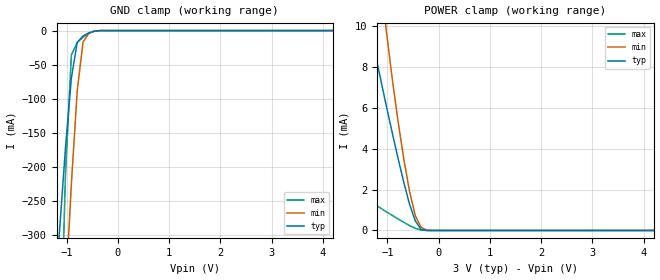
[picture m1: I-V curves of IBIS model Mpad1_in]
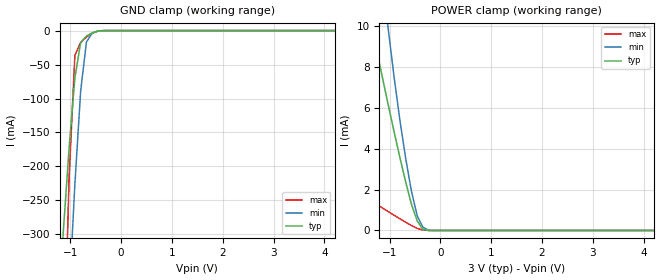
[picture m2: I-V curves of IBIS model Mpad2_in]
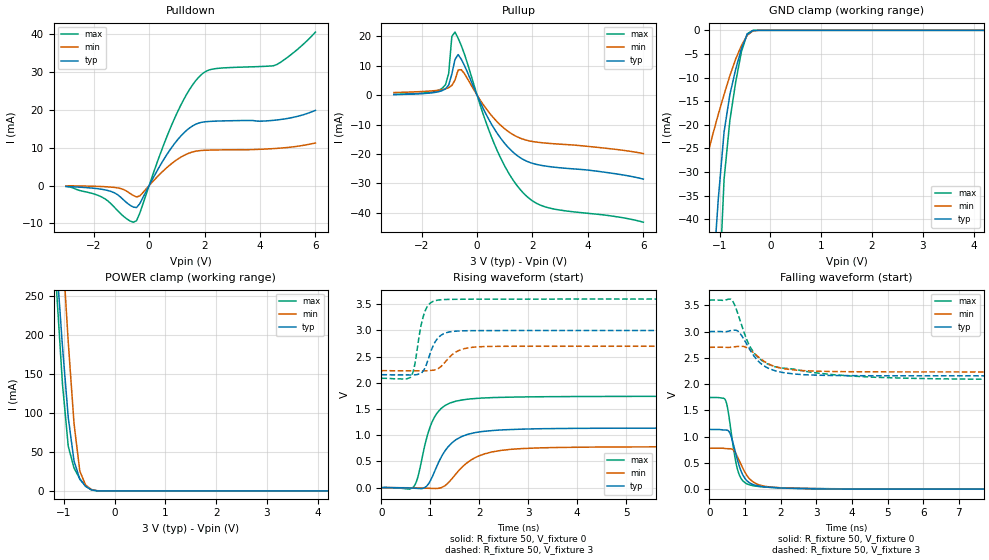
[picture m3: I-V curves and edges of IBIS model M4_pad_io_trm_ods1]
| Created by SiliconSmart  O-2018.09-SP2-3
[IBIS Ver]   4.0
[File Name]   as3316tb_rev1p3.ibs
[File Rev]   1.3
[Date]   Thursday Mar 21 2024
|[Source]   Avalanche Team
|[Notes]   Generated IBIS models from Silicon Smart
|[Rev 1.0]  Initial Release based on extracted netlist
|   Characterization
|[Rev 1.1]  Recharacterization with Hspice, run in high accuracy mode
|[Rev 1.2]  Recharacterization with Hspice, align with parameters
|   in datasheet rev T
|[Rev 1.3]  Update the pin to the package pinout assignment
|[Disclaimer]   THE MODEL LIBRARIES ARE PROVIDED AS IS.
|[Copyright]   Copyright 2019, Avalanche Technology., All Rights Reserved
[Component]   as30xx316_TSOP54
[Manufacturer] Avalanche Technology
| CONTENT :
| This file contains IBIS MODEL for PSRAM device
| AS3032316
| USAGE :
| The models are derived for the 2.7V to 3.6V I/O Operation.
| Temperatures for model generation: typ: 25, max: -40, min: 105
| Voltages : typ: 3.0V, min: 2.7V, max: 3.6V
| PACKAGES SUPPORTED :
| 54-pin TSOP (10mm x 22mm)
| VERIFICATION
| Errors  : 0
| Warnings: 11
| All warnings due to non-monotonic data:
[Package]
R_pkg   0   0 0
L_pkg   0   0 0
C_pkg   0   0 0
[Pin]   signal_name   model_name R_pin   L_pin   C_pin
1   ADDR_20   Mpad1_in   0.242	9.288E-9	1.318E-12
2   ADDR_19   Mpad1_in   0.230	8.645E-9	1.393E-12
3   ADDR_0   Mpad1_in   0.220	8.000E-9	1.249E-12
4   ADDR_1   Mpad1_in   0.202	7.235E-9	1.120E-12
5   ADDR_2   Mpad1_in   0.190	6.504E-9	9.932E-13
6   ADDR_3   Mpad1_in   0.183	5.790E-9	7.992E-13
7   ADDR_4   Mpad1_in   0.153	4.971E-9	7.183E-13
8   E#   Mpad2_in   0.144	4.305E-9	7.146E-13
9   DQ_0   Mpad_io   0.133	3.895E-9	6.207E-13
10   DQ_1   Mpad_io   0.123	3.499E-9	5.802E-13
11   DQ_2   Mpad_io   0.118	3.169E-9	5.261E-13
12   DQ_3   Mpad_io   0.114	2.900E-9	4.467E-13
15   DQ_4   Mpad_io   0.109	2.671E-9	4.016E-13
16   DQ_5   Mpad_io   0.111	2.843E-9	4.439E-13
17   DQ_6   Mpad_io   0.114	3.087E-9	5.185E-13
18   DQ_7   Mpad_io   0.118	3.390E-9	5.728E-13
19   W#   Mpad2_in   0.125	3.746E-9	6.059E-13
20   ADDR_5   Mpad1_in   0.134	4.125E-9	6.880E-13
21   ADDR_6   Mpad1_in   0.156	5.043E-9	7.141E-13
22   ADDR_7   Mpad1_in   0.191	5.914E-9	8.117E-13
23   ADDR_8   Mpad1_in   0.203	6.653E-9	1.003E-12
24   ADDR_9   Mpad1_in   0.215	7.410E-9	1.094E-12
31   ADDR_10   Mpad1_in   0.215	7.409E-9	1.099E-12
32   ADDR_11   Mpad1_in   0.202	6.635E-9	1.007E-12
33   ADDR_12   Mpad1_in   0.190	5.904E-9	8.154E-13
34   ADDR_13   Mpad1_in   0.155	5.033E-9	7.165E-13
35   ADDR_14   Mpad1_in   0.134	4.125E-9	6.860E-13
37   DQ_8   Mpad_io   0.118	3.397E-9	5.722E-13
38   DQ_9   Mpad_io   0.114	3.090E-9	5.214E-13
39   DQ_10   Mpad_io   0.111	2.837E-9	4.444E-13
40   DQ_11   Mpad_io   0.109	2.663E-9	4.035E-13
43   DQ_12   Mpad_io   0.114	2.913E-9	4.507E-13
44   DQ_13   Mpad_io   0.118	3.178E-9	5.252E-13
45   DQ_14   Mpad_io   0.123	3.501E-9	5.817E-13
46   DQ_15   Mpad_io   0.133	3.900E-9	6.217E-13
47   LB#   Mpad2_in   0.143	4.301E-9	7.117E-13
48   UB#   Mpad2_in   0.153	4.972E-9	7.207E-13
49   G#   Mpad2_in   0.179	5.774E-9	7.991E-13
50   ADDR_15   Mpad1_in   0.191	6.496E-9	9.963E-13
51   ADDR_16   Mpad1_in   0.204	7.263E-9	1.127E-12
52   ADDR_17   Mpad1_in   0.221	8.012E-9	1.250E-12
53   ADDR_18   Mpad1_in   0.232	8.680E-9	1.364E-12
13   VCC   POWER   NA   NA   NA
14   VSS   GND   NA   NA   NA
41   VCC   POWER   NA   NA   NA
42   VSS   GND   NA   NA   NA
| pad_io
[Model Selector] Mpad_io
| Model Description
M4_pad_io_trm_ods1   60 Ohms drv strength
| Models and submodels in the file (3): Mpad1_in (Input), Mpad2_in (Input), M4_pad_io_trm_ods1 (I/O)
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| pad1_in
[Model] Mpad1_in
Model_type Input
Enable   Active-High
Vinl  =  0.6
Vinh  =  2.4
| Capacitance  typ   min   max
C_comp   2.857182e-12   2.353202e-12   3.152994e-12
| Variables   typ   min   max
[GND Clamp Reference]   0   0   0
[POWER Clamp Reference]   3   2.7   3.6
[Pulldown Reference]   0   0   0
[Pullup Reference]   3   2.7   3.6
[Temperature Range]   25   105   -40
[Voltage Range]   3   2.7   3.6
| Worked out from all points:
|   GND clamp passes 1 mA (typ) near -0.47 V on its own axis
|   POWER clamp passes 1 mA (typ) near -0.53 V on its own axis
[GND Clamp]
| Voltage   I(typ)   I(min)   I(max)
-3V       -2.489A    -3.622A    -6.286A
-1.252V   -415.1mA   -737.7mA   -841.9mA
-1.138V   -289.6mA   -559.5mA   -509.9mA
-1.024V   -170.9mA   -387mA     -208.5mA
-910.3mV  -69.58mA   -225.3mA   -35.91mA
-796.6mV  -17.5mA    -88.85mA   -17.44mA
-682.8mV  -8.077mA   -16.84mA   -9.651mA
-569mV    -3.425mA   -3.886mA   -3.679mA
-455.2mV  -663.4uA   -928.9uA   -526.9uA
-227.6mV  -421.5nA   -3.52uA    -35.99nA
6V        0A         0A         0A
[POWER Clamp]
| Voltage   I(typ)   I(min)   I(max)
-3V       32.41mA    56.72mA    4.109mA
-1.366V   10.2mA     17.4mA     1.461mA
-1.252V   8.822mA    14.8mA     1.281mA
-1.024V   6.137mA    9.837mA    922.9uA
-910.3mV  4.838mA    7.526mA    746.6uA
-796.6mV  3.581mA    5.417mA    573.1uA
-682.8mV  2.387mA    3.545mA    403.9uA
-569mV    1.291mA    1.93mA     242.9uA
-455.2mV  467.9uA    721.2uA    103.5uA
-341.4mV  48.97uA    156.2uA    20.84uA
-113.8mV  7.993nA    354.4nA    880.4pA
6V        0A         0A         0A
| pad2_in
[Model] Mpad2_in
Model_type Input
Enable   Active-High
Vinl  =  0.6
Vinh  =  2.4
| Capacitance  typ   min   max
C_comp   2.865723e-12   2.362138e-12   3.161751e-12
| Variables   typ   min   max
[GND Clamp Reference]   0   0   0
[POWER Clamp Reference]   3   2.7   3.6
[Pulldown Reference]   0   0   0
[Pullup Reference]   3   2.7   3.6
[Temperature Range]   25   105   -40
[Voltage Range]   3   2.7   3.6
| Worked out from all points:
|   GND clamp passes 1 mA (typ) near -0.47 V on its own axis
|   POWER clamp passes 1 mA (typ) near -0.53 V on its own axis
[GND Clamp]
| Voltage   I(typ)   I(min)   I(max)
-3V       -2.583A    -3.873A    -6.564A
-1.138V   -296.1mA   -573.1mA   -531mA
-1.024V   -173.3mA   -391.8mA   -216.6mA
-910.3mV  -69.77mA   -226.3mA   -36.44mA
-796.6mV  -17.49mA   -89.03mA   -17.43mA
-682.8mV  -8.073mA   -16.84mA   -9.646mA
-569mV    -3.423mA   -3.884mA   -3.677mA
-455.2mV  -662.9uA   -928.4uA   -526.4uA
-227.6mV  -421nA     -3.517uA   -35.92nA
6V        0A         0A         0A
[POWER Clamp]
| Voltage   I(typ)   I(min)   I(max)
-3V       32.41mA    56.72mA    4.109mA
-1.366V   10.2mA     17.4mA     1.461mA
-1.252V   8.822mA    14.8mA     1.281mA
-1.024V   6.137mA    9.837mA    922.9uA
-910.3mV  4.838mA    7.526mA    746.6uA
-796.6mV  3.581mA    5.417mA    573.1uA
-682.8mV  2.387mA    3.545mA    403.9uA
-569mV    1.291mA    1.93mA     242.9uA
-455.2mV  467.9uA    721.2uA    103.5uA
-341.4mV  48.97uA    156.2uA    20.84uA
-113.8mV  7.993nA    354.4nA    880.4pA
6V        0A         0A         0A
[Model] M4_pad_io_trm_ods1
Model_type I/O
Enable   Active-High
Vinl  =  0.6
Vinh  =  2.4
Vmeas =  1.5
Cref  =  30e-12
| Capacitance  typ   min   max
C_comp   4.118801e-12   3.947848e-12   4.414159e-12
| Variables   typ   min   max
[GND Clamp Reference]   0   0   0
[POWER Clamp Reference]   3   2.7   3.6
[Pulldown Reference]   0   0   0
[Pullup Reference]   3   2.7   3.6
[Temperature Range]   25   105   -40
[Voltage Range]   3   2.7   3.6
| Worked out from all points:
|   slope of the pulldown table from 0 to 0.45 V, typ, clamps not added: 75.6 ohm
|   slope of the pullup table from 0 to 0.45 V, typ, clamps not added: 51.8 ohm
|   GND clamp passes 1 mA (typ) near -0.46 V on its own axis
|   POWER clamp passes 1 mA (typ) near -0.42 V on its own axis
|   falling waveform, R_fixture 50, V_fixture 0: 20-80 % time 325ps typ, 411ps min, 252ps max; typ from 1.14 V to 0 V
|   falling waveform, R_fixture 50, V_fixture 3: 20-80 % time 602ps typ, 661ps min, 794ps max; typ from 3 V to 2.15 V
|   rising waveform, R_fixture 50, V_fixture 0: 20-80 % time 466ps typ, 621ps min, 335ps max; typ from 0 V to 1.14 V
|   rising waveform, R_fixture 50, V_fixture 3: 20-80 % time 225ps typ, 326ps min, 176ps max; typ from 2.15 V to 3 V
[GND Clamp]
| Voltage   I(typ)   I(min)   I(max)
-3V       -379.8mA   -106mA     -725.8mA
-1.593V   -131.7mA   -42.01mA   -247mA
-1.479V   -111.8mA   -36.94mA   -208.5mA
-1.138V   -53.52mA   -22.25mA   -94.22mA
-1.024V   -35.67mA   -17.76mA   -59.08mA
-910.3mV  -21.49mA   -13.58mA   -31.51mA
-796.6mV  -13.6mA    -9.604mA   -19.09mA
-682.8mV  -8.279mA   -6.099mA   -11mA
-569mV    -3.88mA    -3.236mA   -4.53mA
-455.2mV  -866.7uA   -1.043mA   -727.1uA
-341.4mV  -35.72uA   -109.2uA   -11.2uA
6V        0A         0A         0A
[POWER Clamp]
| Voltage   I(typ)   I(min)   I(max)
-3V       2.191A     2.679A     2.475A
-1.138V   291mA      439mA      255.8mA
-1.024V   186.1mA    312.2mA    137.6mA
-910.3mV  94.47mA    191.5mA    57.5mA
-796.6mV  38.47mA    86.67mA    29.42mA
-682.8mV  15.04mA    25.47mA    15.61mA
-569mV    5.939mA    7.524mA    6.125mA
-455.2mV  1.483mA    1.86mA     1.35mA
-227.6mV  1.148uA    12.93uA    332nA
6V        0A         0A         0A
[Pulldown]
| Voltage   I(typ)   I(min)   I(max)
-3V       -248.9uA   -57.27uA   -211.8uA
-1.934V   -763.9uA   -203.6uA   -2.351mA
-1.479V   -1.326mA   -352.6uA   -4.122mA
-796.6mV  -4.614mA   -1.551mA   -8.859mA
-455.2mV  -5.81mA    -3.008mA   -9.281mA
413.8mV   5.511mA    3.198mA    8.617mA
827.6mV   10.2mA     5.892mA    16.24mA
1.345V    14.53mA    8.266mA    23.98mA
1.759V    16.42mA    9.161mA    28.37mA
2.276V    16.97mA    9.375mA    30.72mA
4.614V    17.32mA    9.818mA    31.97mA
6V        19.86mA    11.25mA    40.51mA
[Pullup]
| Voltage   I(typ)   I(min)   I(max)
-3V       187.4uA    871.4uA    220.3uA
-1.252V   1.555mA    1.876mA    2.377mA
-1.024V   3.43mA     2.541mA    7.364mA
-910.3mV  7.139mA    3.267mA    19.92mA
-796.6mV  12.13mA    5.096mA    21.41mA
-682.8mV  13.76mA    8.544mA    19.32mA
-569mV    12.16mA    8.636mA    16.81mA
620.7mV   -11.43mA   -8.01mA    -16.55mA
1.138V    -17.91mA   -12.44mA   -26.44mA
1.655V    -21.81mA   -14.96mA   -33.11mA
2.586V    -24.25mA   -16.39mA   -38.3mA
6V        -28.52mA   -19.85mA   -43.17mA
[Ramp]
dV/dt_r   0.681951/0.465717n  0.468514/0.620601n  1.04707/0.335033n
dV/dt_f   0.507478/0.602469n  0.281038/0.661038n  0.908676/0.793971n
R_load = 50
[Falling Waveform]
R_fixture = 50
V_fixture = 0
V_fixture_min = 0
V_fixture_max = 0
| Time   V(typ)   V(min)   V(max)
0s        1.137V     780.9mV    1.745V
449.9ps   1.126V     772.6mV    1.697V
508.1ps   1.122V     771mV      1.558V
603.1ps   1.02V      768.8mV    1.127V
721ps     726.5mV    702.8mV    590.2mV
828.5ps   459.1mV    557.6mV    291.5mV
1.004ns   198.3mV    313.9mV    120.4mV
1.349ns   64.63mV    94.58mV    52.82mV
3.774ns   2.102mV    4.005mV    6.578mV
21.88ns   -42.85nV   140nV      61.39nV
[Falling Waveform]
R_fixture = 50
V_fixture = 3
V_fixture_min = 2.7
V_fixture_max = 3.6
| Time   V(typ)   V(min)   V(max)
0s        3V         2.7V       3.6V
634.8ps   3.023V     2.703V     3.597V
847.3ps   2.977V     2.719V     3.241V
1.169ns   2.619V     2.638V     2.678V
1.378ns   2.432V     2.516V     2.503V
1.62ns    2.314V     2.399V     2.386V
2.203ns   2.207V     2.282V     2.298V
3.494ns   2.163V     2.239V     2.178V
7.486ns   2.158V     2.232V     2.093V
21.88ns   2.154V     2.232V     2.086V
[Rising Waveform]
R_fixture = 50
V_fixture = 0
V_fixture_min = 0
V_fixture_max = 0
| Time   V(typ)   V(min)   V(max)
0s        24.24nV    299.5nV    41.88nV
653.2ps   -9.927mV   -1.656mV   10.12mV
759.1ps   -16.54mV   -3.819mV   256.1mV
919.1ps   24.84mV    -9.607mV   933.3mV
1.136ns   419.1mV    -14.93mV   1.424V
1.43ns    847.3mV    159.7mV    1.625V
1.82ns    1.031V     521.5mV    1.695V
2.443ns   1.101V     711mV      1.724V
3.955ns   1.132V     771.8mV    1.74V
21.88ns   1.137V     780.9mV    1.745V
[Rising Waveform]
R_fixture = 50
V_fixture = 3
V_fixture_min = 2.7
V_fixture_max = 3.6
| Time   V(typ)   V(min)   V(max)
0s        2.154V     2.232V     2.086V
596.6ps   2.152V     2.231V     2.111V
670.7ps   2.154V     2.231V     2.302V
806.3ps   2.186V     2.231V     3.083V
893ps     2.296V     2.231V     3.375V
1.061ns   2.72V      2.243V     3.558V
1.23ns    2.917V     2.326V     3.588V
1.576ns   2.991V     2.616V     3.596V
2.22ns    2.998V     2.696V     3.598V
21.88ns   3V         2.7V       3.6V
